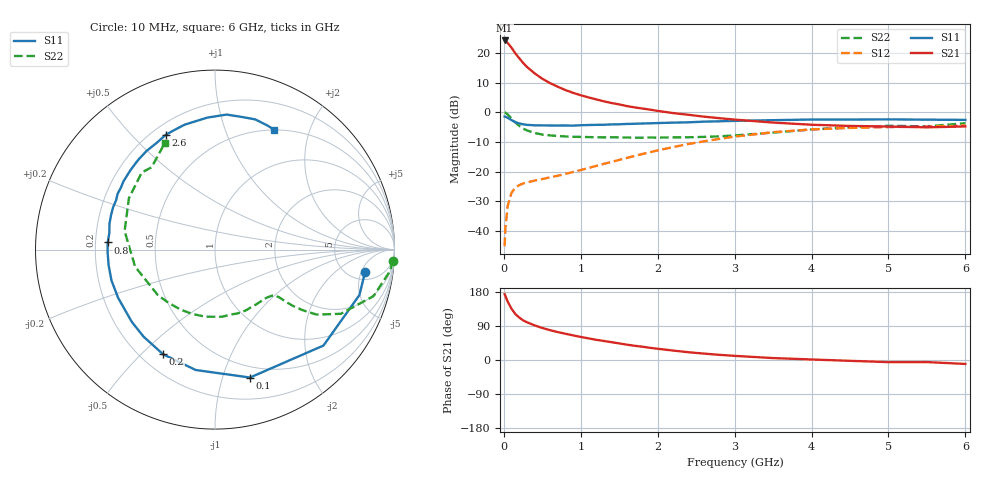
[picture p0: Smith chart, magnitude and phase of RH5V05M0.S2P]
! SIEMENS Small Signal Semiconductors
! BFR106
! Si NPN RF Bipolar Junction Transistor in SOT23
! VCE = 5 V  IC = 5 mA
! Common Emitter S-Parameters:  August  1996
# GHz  S  MA  R  50
!  f  S11  S21  S12  S22
! GHz  MAG  ANG  MAG  ANG  MAG  ANG  MAG  ANG
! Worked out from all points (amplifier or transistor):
!   36 points, 10 MHz to 6 GHz, reference 50 ohm
!   highest |S21| = 24.2 dB at 10 MHz (marker M1)
!   |S21| within 3 dB of that: start of sweep to 114.7 MHz
!   unconditionally stable (mu >= 1): 627.7 MHz to 1.883 GHz; 4.826 GHz to end of sweep
!   at 250 MHz: K = 0.51, MSG = 20.3 dB, |S12| = -23.9 dB
!   at 1.4 GHz: K = 1.13, MAG = 7.7 dB, |S12| = -16.7 dB
!   at 6 GHz: K = 1.02, MAG = -1.0 dB, |S12| = -4.4 dB
!   S11 on the Smith chart (normalised r, x): 10 MHz: 6.65, -5.89; 100 MHz: 0.39, -1.23; 200 MHz: 0.29, -0.58; 800 MHz: 0.25, +0.03; 2.6 GHz: 0.25, +0.63; 6 GHz: 0.50, +1.49
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0.01  0.8454 -8.6  16.13 173.9  0.0056 86.2  0.9933 -3.6
0.02  0.8434 -17.5  15.9 169.2  0.0113 81.0  0.9824 -7.0
0.05  0.8068 -41.5  14.64 154.0  0.0267 69.5  0.9211 -16.3
0.1  0.7389 -74.7  12.18 135.3  0.0443 55.8  0.7876 -27.0
0.15  0.6794 -99.1  9.785 121.1  0.0544 45.9  0.6722 -32.6
0.2  0.6509 -116.4  8.109 112.1  0.0594 42.4  0.5916 -34.7
0.25  0.6273 -129.4  6.778 104.7  0.0635 39.6  0.532 -35.9
0.3  0.6141 -139.0  5.8 99.6  0.066 39.3  0.4961 -36.3
0.4  0.6031 -153.5  4.512 91.4  0.0711 39.9  0.4485 -36.6
0.5  0.6018 -163.5  3.666 84.5  0.0753 42.3  0.4219 -37.3
0.6  0.599 -171.7  3.098 78.8  0.0803 44.9  0.4083 -38.9
0.8  0.5994 176.2  2.365 69.3  0.0919 50.7  0.3924 -43.3
1.1  0.6103 161.6  1.779 57.1  0.1156 58.1  0.3825 -52.3
1.3  0.6156 153.6  1.528 50.2  0.1357 61.3  0.3787 -59.2
1.6  0.6361 143.3  1.27 40.4  0.1709 63.6  0.3768 -71.0
2.2  0.6692 124.6  0.97 24.9  0.2598 61.2  0.3779 -98.2
2.6  0.6958 113.2  0.844 16.9  0.3244 55.8  0.3854 -119.5
3.5  0.7365 93.4  0.671 5.1  0.4623 39.2  0.4553 -168.0
4.5  0.7541 78.4  0.589 -2.2  0.5454 19.2  0.5585 149.2
5  0.7593 72.8  0.575 -5.6  0.5638 10.9  0.5925 133.5
5.5  0.7507 67.2  0.558 -5.5  0.5724 6.7  0.5788 127.6
6  0.7452 63.7  0.578 -10.4  0.6009 -1.4  0.655 115.4
